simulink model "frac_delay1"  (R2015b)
settings: Solver=VariableStepAuto  StartTime=0.0  StopTime=10.0  RelTol=1e-3
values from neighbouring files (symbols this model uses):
  delay1 = D*10    (= 46)    [frac_delay_1.m]    (also in frac_delay_2.m = 116)
  h = sinc(n-D)    [frac_delay_0.m]    (also in frac_delay_1.m = h.*hanning(length(h))'; frac_delay_2.m = h.*hanning(length(h))'; ifir_1.m = firpm(nord_exp,[0,fp*L,fs*L,0.5]*2,[1,1,0,0],[1,10]); ifir_dezim_1.m = firpm(nord_exp,[0,fp*L,fsp*L,0.5]*2,[1,1,0,0],[1,10]))
  hTP = fir1(nord, 2*fp/fs)    [dezimier_2.m]    (also in dezimier_3.m; frac_delay_1.m = fir1(nord, fp*2); frac_delay_2.m = fir1(nord, fp*2); lagrange_3.m = fir1(40, 0.5))
  Ts = 1/fs    (= 5e-05)    [basisband_1.m]    (also in basisband_2.m = 5e-06; dezimier_1.m = 0.0005; dezimier_11.m = 0.0005; dezimier_2.m = 0.0005)
  Ts1 = Ts/10    (= 0.01)    [frac_delay_1.m]    (also in frac_delay_2.m; abtast_rate_1.m = 0.001)
libraries: simulink x1

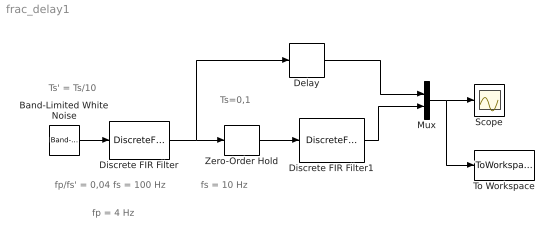
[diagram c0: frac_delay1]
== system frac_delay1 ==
  note: fs = 10 Hz
  note: fp = 4 Hz
  note: fp/fs' = 0,04 fs = 100 Hz
  note: Ts=0,1
  note: Ts' = Ts/10
  Band-Limited White Noise : simulink/Sources/Band-Limited White Noise  Cov=Ts/10  Ts=Ts1  seed=[23341]
  Delay : Delay  DelayLength=delay1
  Discrete FIR Filter : DiscreteFir  Coefficients=hTP  SampleTime=Ts1
  Discrete FIR Filter1 : DiscreteFir  Coefficients=h  SampleTime=Ts
  Mux : Mux  Inputs=2
  Scope : Scope
  To Workspace : ToWorkspace  VariableName=y  SaveFormat=Timeseries  SampleTime=-1
  Zero-Order Hold : ZeroOrderHold  SampleTime=Ts
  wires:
  Band-Limited White Noise/1 -> Discrete FIR Filter/1
  Mux/1 -> Scope/1, To Workspace/1
  Discrete FIR Filter/1 -> Delay/1, Zero-Order Hold/1
  Delay/1 -> Mux/1
  Zero-Order Hold/1 -> Discrete FIR Filter1/1
  Discrete FIR Filter1/1 -> Mux/2
